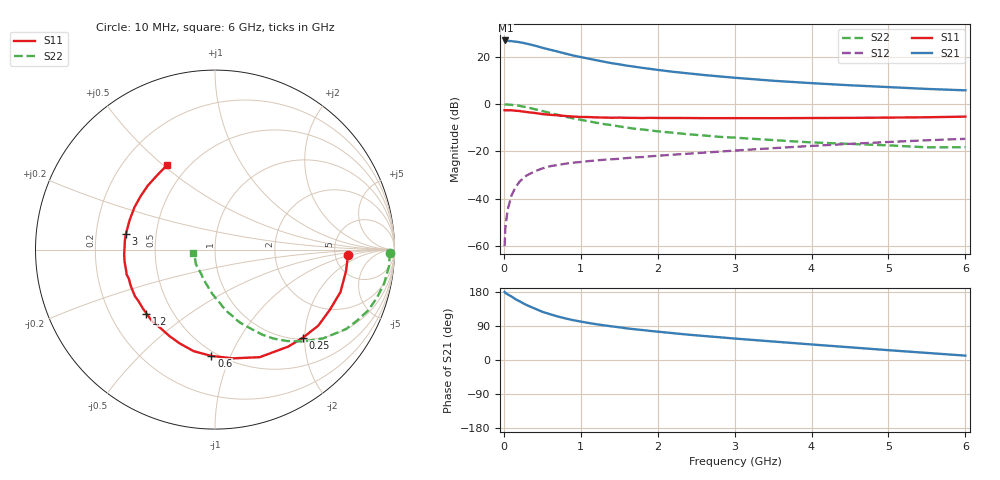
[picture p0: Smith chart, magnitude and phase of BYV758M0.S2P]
! SIEMENS Small Signal Semiconductors
! BFY420
! Si NPN RF SIEGET Grounded Emitter Transistor in MICRO-X
! VCE = 0.75 V  IC = 8 mA
! Common Emitter S-Parameters:  October  1996
# GHz  S  MA  R  50
!  f  S11  S21  S12  S22
! GHz  MAG  ANG  MAG  ANG  MAG  ANG  MAG  ANG
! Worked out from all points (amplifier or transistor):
!   36 points, 10 MHz to 6 GHz, reference 50 ohm
!   highest |S21| = 26.8 dB at 20 MHz (marker M1)
!   |S21| within 3 dB of that: start of sweep to 490.4 MHz
!   unconditionally stable (mu >= 1): 2.535 GHz to end of sweep
!   at 250 MHz: K = 0.17, MSG = 28.6 dB, |S12| = -31.3 dB
!   at 1.4 GHz: K = 0.71, MSG = 20.3 dB, |S12| = -23.3 dB
!   at 6 GHz: K = 1.14, MAG = 8.0 dB, |S12| = -14.7 dB
!   S11 on the Smith chart (normalised r, x): 10 MHz: 6.63, -0.88; 250 MHz: 1.03, -1.95; 600 MHz: 0.47, -0.85; 1.2 GHz: 0.36, -0.35; 3 GHz: 0.33, +0.08; 6 GHz: 0.39, +0.52
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0.01  0.7418 -2.3  21.94 179.6  0.001 92.7  0.9747 -1.0
0.02  0.7403 -4.1  21.98 177.0  0.0025 88.9  0.9739 -2.1
0.1  0.738 -18.7  21.25 167.7  0.0118 80.7  0.9613 -11.2
0.15  0.7225 -27.8  20.75 160.6  0.0173 75.2  0.9408 -16.7
0.2  0.7144 -36.4  20.24 155.6  0.0225 72.3  0.9178 -21.7
0.25  0.6932 -45.2  19.52 149.7  0.0271 68.1  0.8842 -26.7
0.3  0.677 -53.0  18.75 144.6  0.0313 64.7  0.8542 -31.2
0.4  0.6492 -67.4  17.16 135.9  0.0379 59.1  0.7806 -39.3
0.5  0.6139 -80.7  15.4 127.3  0.0437 54.2  0.7117 -46.0
0.6  0.5928 -91.9  14.05 120.9  0.0487 50.5  0.6491 -51.7
0.7  0.5784 -101.8  12.82 114.8  0.0517 47.9  0.593 -56.7
0.8  0.5585 -110.6  11.62 109.7  0.055 45.4  0.5425 -60.9
0.9  0.5447 -117.7  10.61 105.2  0.0579 43.5  0.4985 -64.3
1.1  0.5313 -131.3  9.096 97.7  0.0624 42.0  0.4327 -70.8
1.2  0.5223 -137.0  8.424 94.5  0.0644 41.2  0.4031 -73.6
1.6  0.5118 -154.6  6.467 83.4  0.0725 39.2  0.3185 -82.6
2.2  0.5083 -172.1  4.794 70.8  0.0853 38.3  0.2483 -93.2
3  0.5044 170.3  3.591 56.6  0.1042 36.4  0.1955 -105.0
3.5  0.5033 160.9  3.103 48.8  0.1171 34.3  0.1734 -112.6
4.5  0.5105 144.0  2.488 33.5  0.1443 28.1  0.144 -128.2
5.5  0.5259 127.1  2.085 18.7  0.1719 20.2  0.1221 -156.2
6  0.5422 119.3  1.947 11.5  0.1844 15.9  0.1226 -172.3
